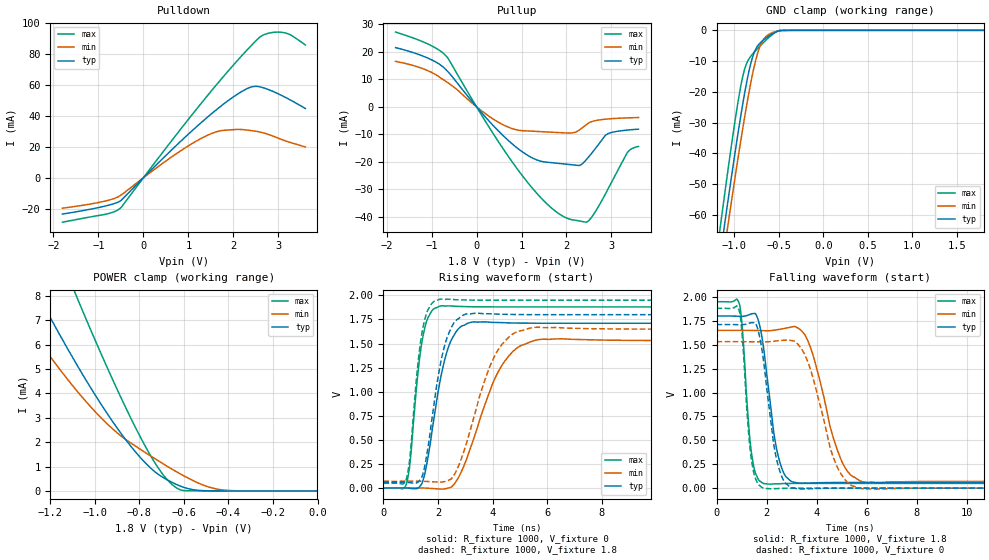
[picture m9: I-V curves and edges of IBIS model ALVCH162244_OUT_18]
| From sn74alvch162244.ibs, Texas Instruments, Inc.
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[Model]   ALVCH162244_OUT_18
Model_type  3-state
Enable   Active-Low
Vref =   0
Rref =   1000
Cref =   30p
Vmeas =   0.9
| variable   typ   min   max
C_comp   7.29pF   6.17pF   8.16pF
| C_pullup   6.44pF   4.68pF   8.53pF
| C_pulldown   5.04pF   4.37pF   5.75pF
| C_tri-state   7.29pF   6.17pF   8.16pF
[Temperature Range]   40   100   -40
| Ambient temperature   25   85   -40
[Voltage range]   1.8   1.65   1.95
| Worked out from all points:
|   slope of the pulldown table from 0 to 0.27 V, typ, clamps not added: 34.4 ohm
|   slope of the pullup table from 0 to 0.27 V, typ, clamps not added: 53.5 ohm
|   GND clamp passes 1 mA (typ) near -0.57 V on its own axis
|   POWER clamp passes 1 mA (typ) near -0.76 V on its own axis
|   rising waveform, R_fixture 1000, V_fixture 0: 20-80 % time 632ps typ, 1.19ns min, 390ps max; typ from 0 V to 1.71 V
|   falling waveform, R_fixture 1000, V_fixture 1.8: 20-80 % time 517ps typ, 925ps min, 308ps max; typ from 1.8 V to 0.059 V
|   rising waveform, R_fixture 1000, V_fixture 1.8: 20-80 % time 592ps typ, 1.06ns min, 382ps max; typ from 0.06 V to 1.8 V
|   falling waveform, R_fixture 1000, V_fixture 0: 20-80 % time 508ps typ, 919ps min, 304ps max; typ from 1.71 V to 0 V
[GND Clamp]
| ALVCH162244_OUT_18
|   Voltage   I(typ)   I(min)   I(max)
-1.8V     -212mA     -215.4mA   -209mA
-1.155V   -72.51mA   -79.89mA   -63.21mA
-1.115V   -64.26mA   -71.86mA   -54.58mA
-1.08V    -57.13mA   -64.9mA    -47.16mA
-1.065V   -54.1mA    -61.94mA   -44.02mA
-960mV    -33.67mA   -41.79mA   -23.46mA
-885mV    -20.5mA    -28.3mA    -12.68mA
-810mV    -10.18mA   -16.26mA   -8.23mA
-740mV    -5.147mA   -7.586mA   -5.932mA
-615mV    -1.896mA   -1.336mA   -2.38mA
-485mV    -30.5uA    -195.8uA   -22.04uA
1.8V      60.47pA    9.424nA    28.01pA
[POWER Clamp]
| ALVCH162244_OUT_18
|   Voltage   I(typ)   I(min)   I(max)
-1.8V     18.28mA    14.1mA     25.42mA
-1.405V   10.7mA     8.206mA    15.46mA
-1.37V    10.07mA    7.723mA    14.62mA
-1.24V    7.782mA    6.003mA    11.54mA
-1.09V    5.319mA    4.207mA    8.149mA
-1.07V    5.007mA    3.987mA    7.711mA
-950mV    3.249mA    2.797mA    5.172mA
-835mV    1.794mA    1.945mA    2.921mA
-725mV    748.5uA    1.292mA    1.078mA
-645mV    315uA      848.1uA    201uA
-435mV    705.1nA    51.1uA     24.09nA
-16.28fV  60.47pA    287pA      33.61pA
[Pulldown]
| ALVCH162244_OUT_18
|   Voltage   I(typ)   I(min)   I(max)
-1.8V     -23.38mA   -19.6mA    -28.64mA
-795mV    -17.84mA   -14.62mA   -23.21mA
-510mV    -14.85mA   -11.36mA   -19.53mA
600mV     17.2mA     12.89mA    22.85mA
1.33V     36.73mA    26.07mA    49.61mA
1.73V     46.37mA    30.4mA     63.6mA
2.335V    57.87mA    30.67mA    83.34mA
2.485V    58.96mA    30.08mA    87.85mA
2.625V    58.35mA    29.27mA    91.4mA
2.935V    54.98mA    26.27mA    93.89mA
3.24V     50.58mA    23mA       92.54mA
3.6V      44.64mA    19.93mA    85.65mA
[Pullup]
| ALVCH162244_OUT_18
|   Voltage   I(typ)   I(min)   I(max)
-1.8V     21.53mA    16.55mA    27.19mA
-1.145V   18.16mA    13.58mA    23.33mA
-685mV    13.61mA    9.278mA    18.65mA
300mV     -5.582mA   -3.69mA    -7.96mA
900mV     -14.94mA   -8.425mA   -22.47mA
1.38V     -19.57mA   -8.997mA   -32.21mA
1.975V    -20.85mA   -9.505mA   -40.28mA
2.295V    -21.31mA   -8.315mA   -41.58mA
2.495V    -18.2mA    -5.869mA   -41.41mA
2.905V    -9.934mA   -4.444mA   -30.48mA
3.355V    -8.465mA   -4.028mA   -16.63mA
3.6V      -8.145mA   -3.908mA   -14.43mA
[Ramp]
| ALVCH162244_OUT_18
| variable   typ   min   max
dV/dt_r   1.04/6.63E-10   0.93/1.27E-09   1.14/4.15E-10
dV/dt_f   1.06/5.69E-10   0.98/1.03E-09   1.16/3.24E-10
R_load = 1000
[Rising Waveform]
| ALVCH162244_OUT_18
R_fixture =   1000
C_fixture =   0
L_fixture =   0
V_fixture =   0
V_fixture_min = 0
V_fixture_max = 0
|   Time   V(typ)   V(min)   V(max)
0s        201uV      221.9uV    178.7uV
850ps     774uV      1.101mV    51.56mV
1.41ns    46.99mV    1.02mV     1.516V
1.65ns    348.8mV    -1.56mV    1.78V
2.105ns   1.156V     -10.23mV   1.891V
2.44ns    1.508V     5.482mV    1.891V
2.865ns   1.681V     178.2mV    1.885V
4.295ns   1.718V     1.254V     1.881V
5.7ns     1.711V     1.542V     1.881V
40ns      1.711V     1.532V     1.881V
[Falling Waveform]
| ALVCH162244_OUT_18
R_fixture =   1000
C_fixture =   0
L_fixture =   0
V_fixture =   1.8
V_fixture_min = 1.65
V_fixture_max = 1.95
|   Time   V(typ)   V(min)   V(max)
0s        1.8V       1.65V      1.95V
930ps     1.797V     1.65V      1.912V
1.395ns   1.823V     1.649V     370.5mV
1.905ns   1.418V     1.647V     47.03mV
2.34ns    496.6mV    1.653V     44.44mV
2.77ns    121mV      1.673V     48.07mV
3.57ns    52.97mV    1.585V     49.57mV
4.95ns    59.46mV    315.6mV    49.21mV
5.945ns   59.61mV    59.33mV    49.23mV
40ns      59.49mV    70.7mV     49.27mV
[Rising Waveform]
| ALVCH162244_OUT_18
R_fixture =   1000
C_fixture =   0
L_fixture =   0
V_fixture =   1.8
V_fixture_min = 1.65
V_fixture_max = 1.95
|   Time   V(typ)   V(min)   V(max)
0s        59.69mV    70.92mV    49.45mV
845ps     59.81mV    71.73mV    99.16mV
1.405ns   111.8mV    70.68mV    1.6V
1.64ns    436.8mV    68.2mV     1.855V
2.09ns    1.291V     62.27mV    1.961V
2.47ns    1.657V     92.1mV     1.96V
2.925ns   1.796V     363.5mV    1.953V
4.115ns   1.806V     1.394V     1.95V
5.46ns    1.8V       1.665V     1.95V
40ns      1.8V       1.65V      1.95V
[Falling Waveform]
| ALVCH162244_OUT_18
R_fixture =   1000
C_fixture =   0
L_fixture =   0
V_fixture =   0
V_fixture_min = 0
V_fixture_max = 0
|   Time   V(typ)   V(min)   V(max)
0s        1.711V     1.532V     1.88V
930ps     1.709V     1.532V     1.834V
1.385ns   1.731V     1.531V     314.7mV
1.885ns   1.319V     1.531V     518uV
2.315ns   415.3mV    1.537V     -5.027mV
2.735ns   58.14mV    1.548V     -1.665mV
3.59ns    -7.07mV    1.36V      183.7uV
4.885ns   -162.1uV   190mV      -38.62uV
5.82ns    125.2uV    -7.025mV   -31.89uV
40ns      -5.138nV   6.912nV    4.21nV
